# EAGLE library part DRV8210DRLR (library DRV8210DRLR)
Motor / Motion / Ignition Controllers & Drivers 12-V, 1.76-A brushed DC motor driver with auto sleep mode Source: Datasheet
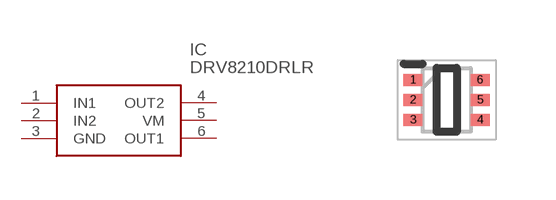
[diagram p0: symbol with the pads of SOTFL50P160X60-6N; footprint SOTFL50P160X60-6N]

Designator prefix IC

## DRV8210DRLR (Description: Motor / Motion / Ignition Controllers & Drivers 12-V, 1.76-A brushed DC motor driver with auto sleep mode; Height: 0.6mm; Manufacturer_Name: Texas Instruments; Manufacturer_Part_Number: DRV8210DRLR; Mouser_Part_Number: 595-DRV8210DRLR; Mouser_Price-Stock: https://www.mouser.co.uk/ProductDetail/Texas-Instruments/DRV8210DRLR?qs=7D1LtPJG0i1B1CHsXZuruQ%3D%3D)  [SOTFL50P160X60-6N]
1  IN1
2  IN2
3  GND
4  OUT2
5  VM
6  OUT1

## Footprint SOTFL50P160X60-6N (pad centres in mm)
DRL (R-PDSO-N6)-
smd 0.475 x 0.3: 1 -0.838,0.5; 2 -0.838,0; 3 -0.838,-0.5; 4 0.838,-0.5; 5 0.838,0; 6 0.838,0.5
